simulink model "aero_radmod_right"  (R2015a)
settings: Solver=ode5  SolverMode=SingleTasking  StartTime=0.0  StopTime=100  FixedStep=0.1  MaxStep=0.1  RelTol=1e-3  AbsTol=1e-6
undefined symbols (not defined in the file): deltat, g, hypot, tauc, tauT
libraries: simulink x2

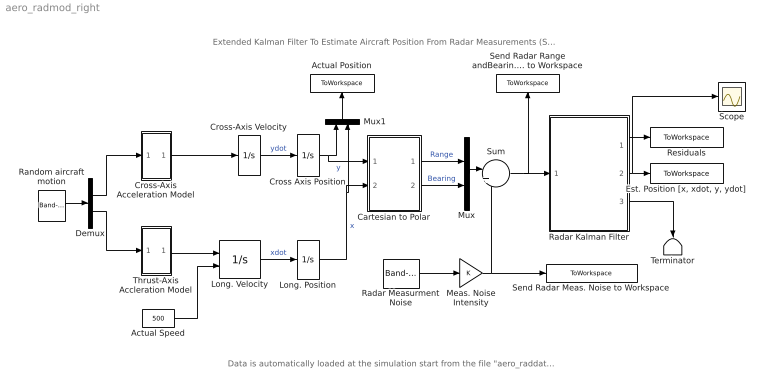
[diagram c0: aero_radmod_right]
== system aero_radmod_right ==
  note: Data is automatically loaded at the simulation start from the file "aero_raddat.m" using an external function call in this model's PreLoadFcn (type 'help set_param' for more info).
  note: Extended Kalman Filter To Estimate Aircraft Position From Radar Measurements (See aero_extkalman.m for implementation of filter)
  Actual Position : ToWorkspace  VariableName=XYCoords
  Actual Speed : Constant  Value=500
  Cartesian to Polar : Subsystem
  "Cross Axis Position " : Integrator
  Cross-Axis Acceleration Model : Subsystem
  Cross-Axis Velocity : Integrator
  Demux : Demux  Outputs=2
  "Est. Position [x, xdot, y, ydot]" : ToWorkspace  VariableName=X_hat  SampleTime=-1
  Long. Position : Integrator
  Long. Velocity : Integrator  InitialConditionSource=external
  Meas. Noise Intensity : Gain
  Mux : Mux  Inputs=2
  Mux1 : Mux  Inputs=2
  Radar Kalman Filter : Subsystem
  Radar Measurment Noise : simulink/Sources/Band-Limited White Noise  Cov=[1 1]  Ts=0.1  seed=[52341 62341]
  Random aircraft motion : simulink/Sources/Band-Limited White Noise  Cov=[0.001 .001]  Ts=0.1  seed=[58413 74925]
  Residuals : ToWorkspace  VariableName=residual  SampleTime=-1
  Scope : Scope
  Send Radar Meas. Noise to Workspace : ToWorkspace  VariableName=Measurement_noise
  Send Radar Range andBearing Angle Meas. to Workspace : ToWorkspace  VariableName=PolarCoords  SampleTime=-1
  Sum : Sum  Inputs=|++
  Terminator : Terminator
  Thrust-Axis Accleration Model : Subsystem
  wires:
  Long. Position/1 -> Mux1/2, Cartesian to Polar/2(y)  "x"
  Cartesian to Polar/2(theta) -> Mux/2  "Bearing"
  Cartesian to Polar/1(r_out) -> Mux/1  "Range"
  Mux/1 -> Sum/1
  Sum/1 -> Radar Kalman Filter/1(Measurements), Send Radar Range andBearing Angle Meas. to Workspace/1
  "Cross Axis Position "/1 -> Mux1/1, Cartesian to Polar/1(x)  "y"
  Cross-Axis Acceleration Model/1(out_1) -> Cross-Axis Velocity/1
  Cross-Axis Velocity/1 -> "Cross Axis Position "/1  "ydot"
  Actual Speed/1 -> Long. Velocity/2
  Long. Velocity/1 -> Long. Position/1  "xdot"
  Thrust-Axis Accleration Model/1(Accleration) -> Long. Velocity/1
  Radar Kalman Filter/1(Resid.) -> Residuals/1
  Demux/1 -> Cross-Axis Acceleration Model/1(Inport)
  Demux/2 -> Thrust-Axis Accleration Model/1(Force)
  Random aircraft motion/1 -> Demux/1
  Mux1/1 -> Actual Position/1
  Radar Measurment Noise/1 -> Meas. Noise Intensity/1
  Meas. Noise Intensity/1 -> Send Radar Meas. Noise to Workspace/1, Sum/2
  Radar Kalman Filter/2(Est. Pos.) -> "Est. Position [x, xdot, y, ydot]"/1, Scope/1
  Radar Kalman Filter/3(Kalman Filter deltat) -> Terminator/1

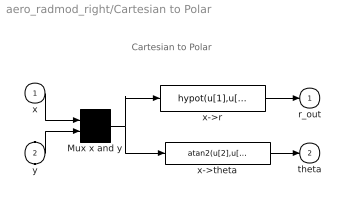
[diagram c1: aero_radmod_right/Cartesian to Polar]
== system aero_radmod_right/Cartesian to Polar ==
  note: Cartesian to Polar
  x : Inport
  y : Inport  Port=2
  Mux x and y : Mux  Inputs=2
  x->r : Fcn  Expr=hypot(u[1],u[2])
  x->theta : Fcn  Expr=atan2(u[2],u[1])
  r_out : Outport
  theta : Outport  Port=2
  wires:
  Mux x and y/1 -> x->r/1, x->theta/1
  x->r/1 -> r_out/1
  x/1 -> Mux x and y/1
  y/1 -> Mux x and y/2
  x->theta/1 -> theta/1

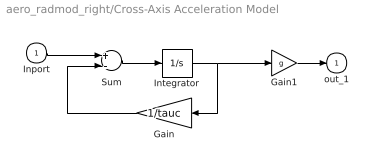
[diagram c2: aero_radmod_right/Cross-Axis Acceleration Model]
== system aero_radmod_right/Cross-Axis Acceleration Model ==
  Inport : Inport
  Gain : Gain  Gain=1/tauc
  Gain1 : Gain  Gain=g
  Integrator : Integrator
  Sum : Sum  Inputs=+-
  out_1 : Outport
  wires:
  Inport/1 -> Sum/1
  Gain/1 -> Sum/2
  Integrator/1 -> Gain1/1, Gain/1
  Sum/1 -> Integrator/1
  Gain1/1 -> out_1/1

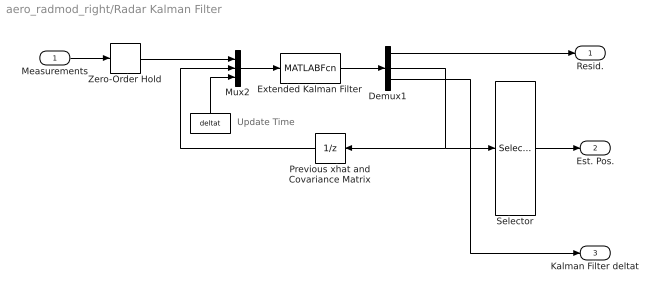
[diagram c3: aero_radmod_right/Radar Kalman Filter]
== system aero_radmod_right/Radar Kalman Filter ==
  note: Update Time
  Measurements : Inport
  " " : Constant  Value=deltat
  Demux1 : Demux  Outputs=[2 20 1]
  Extended Kalman Filter : MATLABFcn  MATLABFcn=aero_extkalman  OutputDimensions=23
  Mux2 : Mux  Inputs=3
  Previous xhat and Covariance Matrix : UnitDelay  InitialCondition=[0.001; 0.01; 0.001; 400; zeros(16,1)]  SampleTime=deltat
  Selector : Selector  InputPortWidth=20  Indices=[1:4]
  Zero-Order Hold : ZeroOrderHold  SampleTime=deltat
  Resid. : Outport
  Est. Pos. : Outport  Port=2
  Kalman Filter deltat : Outport  Port=3
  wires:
  Measurements/1 -> Zero-Order Hold/1
  Extended Kalman Filter/1 -> Demux1/1
  Zero-Order Hold/1 -> Mux2/1
  Selector/1 -> Est. Pos./1
  Demux1/1 -> Resid./1
  Demux1/2 -> Previous xhat and Covariance Matrix/1, Selector/1
  " "/1 -> Mux2/3
  Previous xhat and Covariance Matrix/1 -> Mux2/2
  Mux2/1 -> Extended Kalman Filter/1
  Demux1/3 -> Kalman Filter deltat/1

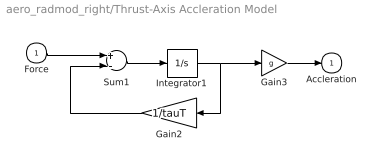
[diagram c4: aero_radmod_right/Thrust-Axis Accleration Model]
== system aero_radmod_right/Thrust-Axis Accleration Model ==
  Force : Inport
  Gain2 : Gain  Gain=1/tauT
  Gain3 : Gain  Gain=g
  Integrator1 : Integrator
  Sum1 : Sum  Inputs=+-
  Accleration : Outport
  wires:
  Force/1 -> Sum1/1
  Gain2/1 -> Sum1/2
  Integrator1/1 -> Gain3/1, Gain2/1
  Sum1/1 -> Integrator1/1
  Gain3/1 -> Accleration/1
